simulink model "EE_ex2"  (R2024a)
settings: Solver=VariableStepAuto  StartTime=0.0  StopTime=70  RelTol=1e-3

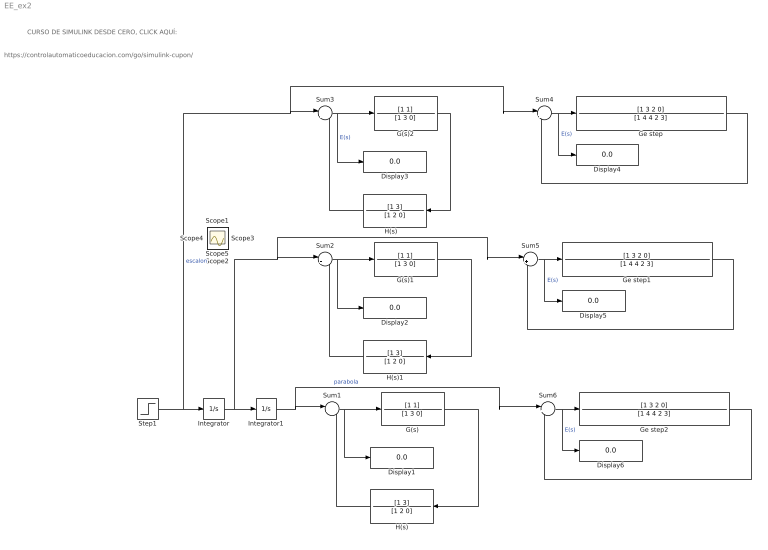
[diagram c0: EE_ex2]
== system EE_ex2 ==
  note: https://controlautomaticoeducacion.com/go/simulink-cupon/
  note: CURSO DE SIMULINK DESDE CERO, CLICK AQUÍ:
  Display{1..6} (6 alike) : Display
  G(s) : TransferFcn  Numerator=[1 1]  Denominator=[1 3 0]
  G(s)1 : TransferFcn  Numerator=[1 1]  Denominator=[1 3 0]
  G(s)2 : TransferFcn  Numerator=[1 1]  Denominator=[1 3 0]
  Ge step : TransferFcn  Numerator=[1 3 2 0]  Denominator=[1 4 4 2 3]
  Ge step1 : TransferFcn  Numerator=[1 3 2 0]  Denominator=[1 4 4 2 3]
  Ge step2 : TransferFcn  Numerator=[1 3 2 0]  Denominator=[1 4 4 2 3]
  H(s) : TransferFcn  Numerator=[1 3]  Denominator=[1 2 0]
  "H(s)    " : TransferFcn  Numerator=[1 3]  Denominator=[1 2 0]
  H(s)1 : TransferFcn  Numerator=[1 3]  Denominator=[1 2 0]
  Integrator : Integrator
  Integrator1 : Integrator
  Step1 : Step  Time=0  SampleTime=0
  Sum{1..6} (6 alike) : Sum  Inputs=|+-
  Scope{,1..5} (6 alike) : Scope
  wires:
  Sum1/1 -> Display1/1, G(s)/1
  H(s)/1 -> Sum1/2
  G(s)/1 -> H(s)/1
  Integrator1/1 -> Sum6/1, Sum1/1  "parabola"
  Step1/1 -> Sum4/1, Sum3/1, Integrator/1  "escalon"
  G(s)1/1 -> H(s)1/1
  H(s)1/1 -> Sum2/2
  Sum2/1 -> G(s)1/1, Display2/1
  Sum3/1 -> Display3/1, G(s)2/1  "E(s)"
  "H(s)    "/1 -> Sum3/2
  G(s)2/1 -> "H(s)    "/1
  Sum4/1 -> Display4/1, Ge step/1  "E(s)"
  Ge step/1 -> Sum4/2
  Ge step1/1 -> Sum5/2
  Sum5/1 -> Ge step1/1, Display5/1  "E(s)"
  Integrator/1 -> Sum5/1, Sum2/1, Integrator1/1
  Sum6/1 -> Display6/1, Ge step2/1  "E(s)"
  Ge step2/1 -> Sum6/2
